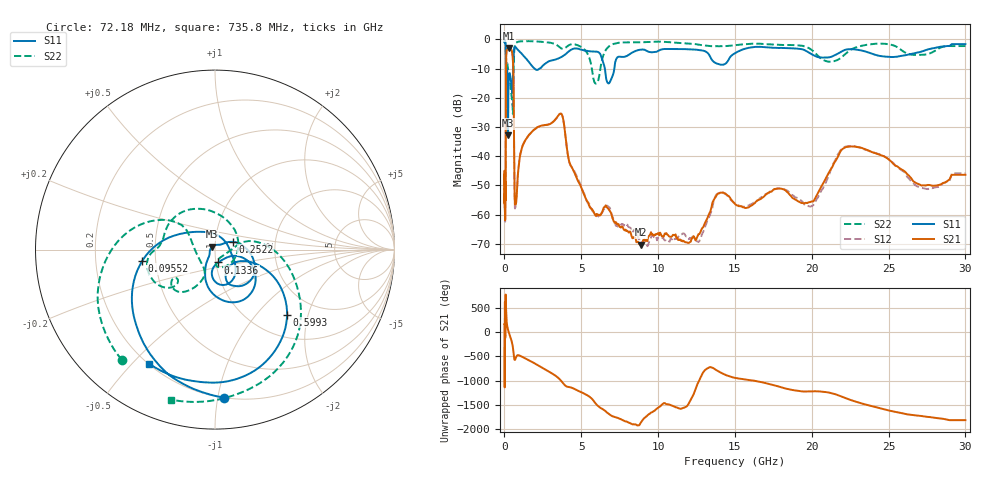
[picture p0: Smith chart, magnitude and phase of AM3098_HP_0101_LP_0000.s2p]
! Date/Time: Thu, Feb 28, 2019 8:35 AM
! Network Analyzer: Agilent Technologies E8364B Rev: A.07.50.67
! Sweep from 0.010 to 30.000 GHz, 1601 Points, Sweep Type: LOG
! Power Supply: 5.023 V, 0.002 A
# Hz S DB R 50
!freq MagS11 AngS11 MagS21 AngS21 MagS12 AngS12 MagS22 AngS22
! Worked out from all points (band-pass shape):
!   1601 points, 10 MHz to 30 GHz, reference 50 ohm
!   highest |S21| = -2.96 dB at 266.5 MHz (marker M1); lowest = -70.3 dB at 8.893 GHz (marker M2)
!   |S21| within 3 dB of the highest: 113.4 MHz to 534.1 MHz (420.7 MHz wide, 130 % of centre)
!   lowest |S11| = -32.8 dB at 230.5 MHz (marker M3), VSWR 1.05, Z = 48.5 + j1.64 ohm
!   |S11| at or under -10 dB: 176.2 MHz to 562.3 MHz (386.1 MHz wide, 105 % of centre); 1.961 GHz to 2.28 GHz (319.6 MHz wide, 15.1 % of centre); 6.533 GHz to 7.149 GHz (615.2 MHz wide, 8.99 % of centre)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
!   |S22| runs from -25.5 to -0.5 dB; largest |S21 - S12| = 0.01
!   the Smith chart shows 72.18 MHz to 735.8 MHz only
!   S11 on the Smith chart (normalised r, x): 72.18 MHz: 0.20, -1.04; 95.52 MHz: 0.42, -0.06; 133.6 MHz: 1.03, -0.15; 252.2 MHz: 1.21, +0.11; 599.3 MHz: 1.45, -1.48; 735.8 MHz: 0.20, -0.56
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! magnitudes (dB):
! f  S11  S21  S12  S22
! 10 MHz  -0.4  -46.3  -46.4  -0.5
! 38.04 MHz  -0.5  -61.3  -57.9  -0.7
! 72.18 MHz  -1.7  -51.7  -54.5  -1.9
! 81.39 MHz  -2.5  -51.3  -48.4  -2.7
! 95.52 MHz  -7.7  -21.5  -21.5  -9.4
! 133.6 MHz  -22.7  -4.1  -4.1  -11.3
! 144.7 MHz  -17.0  -3.7  -3.7  -11.0
! 186.8 MHz  -11.1  -3.5  -3.4  -8.2
! 230.5 MHz  -32.8  -3.1  -3.0  -10.1
! 252.2 MHz  -19.4  -3.0  -2.9  -10.5
! 266.5 MHz  -15.8  -3.0  -2.9  -10.6
! 550.5 MHz  -12.0  -7.2  -7.2  -25.3
! 599.3 MHz  -5.3  -18.4  -18.4  -10.0
! 665.8 MHz  -2.6  -54.5  -55.1  -2.3
! 735.8 MHz  -2.7  -56.0  -56.0  -1.2
! 2.084 GHz  -10.4  -30.3  -30.3  -0.7
! 3.686 GHz  -6.1  -25.4  -25.5  -3.0
! 7.926 GHz  -5.8  -65.7  -63.3  -1.0
! 8.893 GHz  -3.5  -70.3  -69.4  -1.0
! 19.8 GHz  -4.5  -55.8  -57.1  -3.0
! 22.67 GHz  -3.4  -36.7  -36.5  -3.2
! 30 GHz  -1.6  -46.4  -45.8  -2.3
